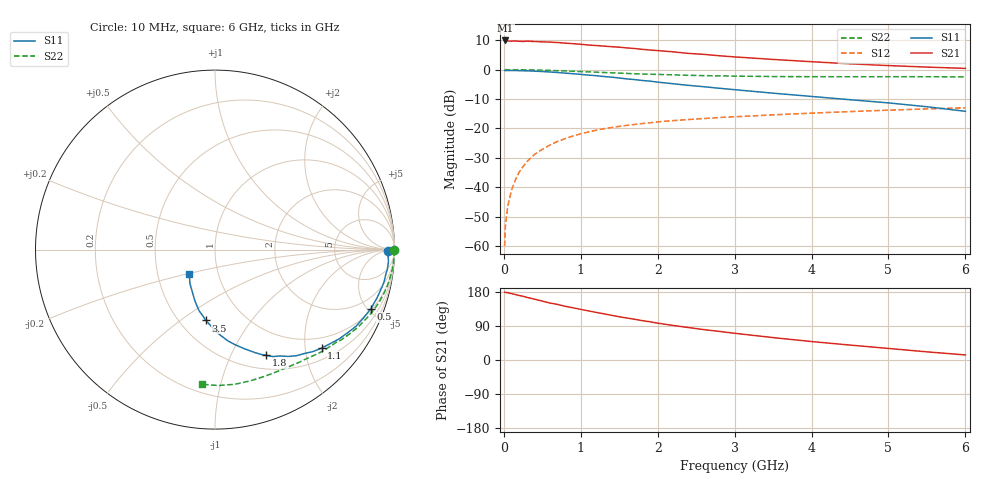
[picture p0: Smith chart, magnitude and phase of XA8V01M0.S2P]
! SIEMENS Discrete & RF Semiconductors
! BFY180
! Si NPN RF Bipolar Junction Transistor in MICRO-X
! VCE = 8 V  IC = 1 mA
! Common Emitter S-Parameters:  May  1997
# GHz  S  MA  R  50
!  f  S11  S21  S12  S22
! GHz  MAG  ANG  MAG  ANG  MAG  ANG  MAG  ANG
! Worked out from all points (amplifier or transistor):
!   36 points, 10 MHz to 6 GHz, reference 50 ohm
!   highest |S21| = 9.9 dB at 20 MHz (marker M1)
!   |S21| within 3 dB of that: start of sweep to 1.793 GHz
!   unconditionally stable (mu >= 1): 4.331 GHz to end of sweep
!   at 250 MHz: K = 0.06, MSG = 21.3 dB, |S12| = -33.0 dB
!   at 1.4 GHz: K = 0.48, MSG = 13.7 dB, |S12| = -19.7 dB
!   at 6 GHz: K = 1.04, MAG = 5.5 dB, |S12| = -13.0 dB
!   S11 on the Smith chart (normalised r, x): 10 MHz: 56, -8; 500 MHz: 1.09, -5.23; 1.1 GHz: 0.74, -2.36; 1.8 GHz: 0.67, -1.37; 3.5 GHz: 0.67, -0.63; 6 GHz: 0.73, -0.20
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0.01  0.9658 -0.3  3.059 178.9  0.001 91.0  0.9983 -0.2
0.02  0.9653 -0.8  3.133 178.4  0.0022 85.1  0.9999 -0.6
0.05  0.9645 -1.9  3.059 177.5  0.0047 82.1  0.9974 -1.3
0.1  0.9686 -3.9  3.048 175.2  0.009 87.8  0.9975 -2.7
0.15  0.9664 -6.5  3.072 172.8  0.0133 87.1  0.9971 -4.0
0.2  0.9616 -8.2  3.031 170.2  0.0182 85.2  0.9958 -5.2
0.3  0.9539 -12.5  3.051 165.2  0.0273 80.3  0.9901 -7.8
0.5  0.9285 -20.8  2.967 155.5  0.0443 75.2  0.9782 -12.8
0.6  0.9104 -24.8  2.938 150.3  0.0525 72.4  0.9695 -15.2
0.7  0.8938 -28.6  2.886 146.6  0.0604 69.4  0.9604 -17.7
0.8  0.872 -32.1  2.819 141.6  0.0675 67.1  0.9499 -20.0
1.1  0.8088 -42.7  2.62 129.6  0.0873 59.8  0.9168 -26.4
1.5  0.7214 -55.6  2.407 114.1  0.1087 51.5  0.8728 -34.1
1.8  0.6542 -64.2  2.213 103.9  0.1214 46.9  0.8433 -39.0
2.2  0.5757 -73.5  2.008 91.2  0.1359 41.1  0.8154 -45.3
2.6  0.5125 -82.1  1.818 80.2  0.1474 36.7  0.7908 -50.7
3  0.4564 -89.4  1.646 70.5  0.158 32.6  0.7756 -55.9
3.5  0.3981 -97.2  1.491 59.1  0.1704 28.4  0.7635 -62.1
4  0.3505 -104.8  1.364 48.7  0.1822 24.2  0.7586 -68.4
4.5  0.3082 -111.2  1.255 39.4  0.1939 20.3  0.7574 -74.9
5.5  0.2341 -126.7  1.105 21.5  0.2151 12.4  0.7575 -88.5
6  0.1959 -136.8  1.05 13.4  0.2245 8.0  0.754 -95.3
